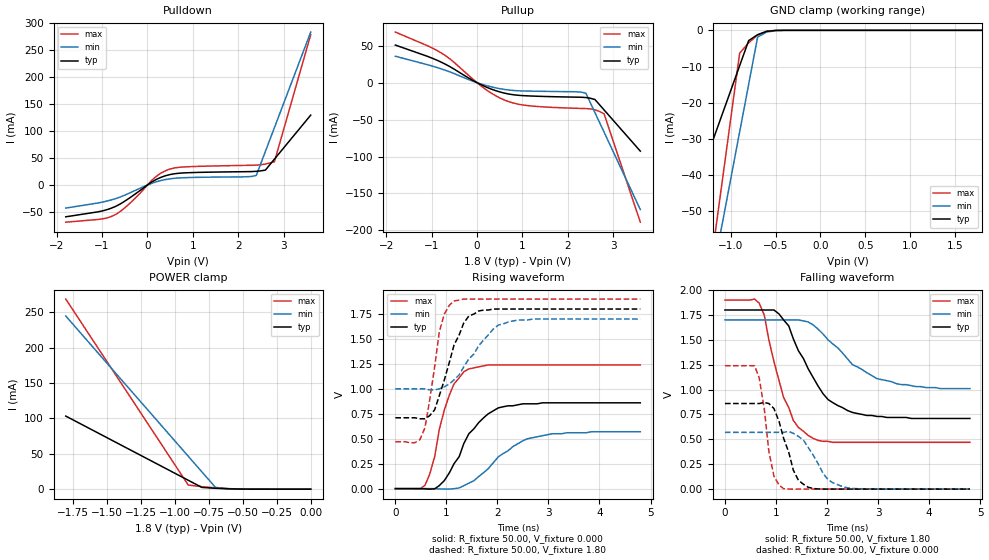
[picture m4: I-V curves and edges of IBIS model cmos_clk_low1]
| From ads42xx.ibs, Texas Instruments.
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|   Model cmos_clk_low1
[Model]   cmos_clk_low1
Model_type   3-state
Polarity   Non-Inverting
Vmeas = 1.0000V
Enable   Active-High
C_comp   5.00pF   2.00pF   8.00pF
[Temperature Range]   25.00   0.12k   -40.00
[Voltage Range]   1.80V   1.70V   1.90V
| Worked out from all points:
|   slope of the pulldown table from 0 to 0.27 V, typ, clamps not added: 20.6 ohm
|   slope of the pullup table from 0 to 0.27 V, typ, clamps not added: 35.4 ohm
|   GND clamp passes 1 mA (typ) near -0.68 V on its own axis
|   POWER clamp passes 1 mA (typ) near -0.67 V on its own axis
|   rising waveform, R_fixture 50.00, V_fixture 0.000: 20-80 % time 614ps typ, 803ps min, 373ps max; typ from 0 V to 0.86 V
|   rising waveform, R_fixture 50.00, V_fixture 1.80: 20-80 % time 423ps typ, 603ps min, 256ps max; typ from 0.71 V to 1.8 V
|   falling waveform, R_fixture 50.00, V_fixture 1.80: 20-80 % time 683ps typ, 937ps min, 475ps max; typ from 1.8 V to 0.71 V
|   falling waveform, R_fixture 50.00, V_fixture 0.000: 20-80 % time 304ps typ, 407ps min, 202ps max; typ from 0.86 V to 0 V
[Pulldown]
| voltage   I(typ)   I(min)   I(max)
-1.8V     -58.78mA   -42.68mA   -68.73mA
-1V       -48.05mA   -31.73mA   -62.68mA
-700mV    -39.48mA   -25.15mA   -54.48mA
-300mV    -18.48mA   -11.25mA   -26.98mA
200mV     10.49mA    6.06mA     16.29mA
500mV     19.33mA    11.46mA    29.59mA
900mV     22.7mA     13.73mA    33.77mA
2.2V      24.65mA    15.28mA    36.32mA
2.4V      25.28mA    17.69mA    36.7mA
2.6V      27.5mA     61.83mA    38.72mA
2.8V      47.82mA    106mA      43mA
3.6V      129.1mA    282.5mA    277.8mA
[Pullup]
| voltage   I(typ)   I(min)   I(max)
-1.8V     50.96mA    35.82mA    68.54mA
-800mV    28.12mA    18.93mA    40.73mA
-600mV    21.83mA    14.64mA    32.36mA
100mV     -3.09mA    -2.01mA    -4.98mA
400mV     -10.58mA   -6.86mA    -17.33mA
600mV     -14.08mA   -9.1mA     -23.36mA
1.1V      -17.8mA    -11.34mA   -30.94mA
2.2V      -19.61mA   -12.37mA   -34.71mA
2.4V      -20.1mA    -14.27mA   -35.09mA
2.6V      -22.83mA   -40.55mA   -36.71mA
2.8V      -36.81mA   -66.83mA   -42.02mA
3.6V      -92.73mA   -171.9mA   -189mA
[GND_clamp]
| voltage   I(typ)   I(min)   I(max)
-1.8V     -72.05mA   -145.9mA   -170.5mA
-1.6V     -58.21mA   -119.7mA   -134mA
-1.5V     -51.29mA   -106.6mA   -115.8mA
-1.2V     -30.53mA   -67.33mA   -61.04mA
-1.1V     -23.61mA   -54.24mA   -42.8mA
-1V       -16.69mA   -41.15mA   -24.56mA
-900mV    -9.77mA    -28.06mA   -6.32mA
-800mV    -2.85mA    -14.97mA   -3.46mA
-700mV    -1.2mA     -1.88mA    -1.32mA
-600mV    -300uA     -470uA     -220uA
-400mV    -2.19uA    -13.33uA   -400nA
1.8V      30.61pA    20.27nA    23.42pA
[POWER_clamp]
| voltage   I(typ)   I(min)   I(max)
-1.8V     103.3mA    244.7mA    268.7mA
-900mV    12.58mA    46.54mA    5.82mA
-800mV    2.5mA      24.52mA    3.54mA
-700mV    1.23mA     2.5mA      1.83mA
-500mV    85.21uA    200uA      92.55uA
0V        30.61pA    840pA      26.65pA
[Ramp]
| variable   typ   min   max
dV/dt_r   0.52/0.58n   0.34/0.80n   0.74/0.39n
dV/dt_f   0.65/0.70n   0.42/0.94n   0.86/0.47n
R_load = 50.00
[Rising Waveform]
R_fixture = 50.00
V_fixture = 0.000
V_fixture_min = 0.000
V_fixture_max = 0.000
| time   V(typ)   V(min)   V(max)
0s        440pV      26.42nV    250pV
580ps     -2.53mV    530uV      33.44mV
770ps     -2.3mV     -810uV     320mV
860ps     30.03mV    -3.05mV    590mV
1.06ns    160mV      -4.45mV    940mV
1.15ns    250mV      -660uV     1.05V
1.44ns    550mV      54.89mV    1.2V
2.02ns    810mV      320mV      1.24V
2.59ns    850mV      500mV      1.24V
4.8ns     860mV      570mV      1.24V
[Rising Waveform]
R_fixture = 50.00
V_fixture = 1.80
V_fixture_min = 1.70
V_fixture_max = 1.90
| time   V(typ)   V(min)   V(max)
0s        710mV      1V         470mV
380ps     710mV      1V         460mV
580ps     700mV      1V         610mV
770ps     790mV      990mV      1.22V
860ps     930mV      1V         1.57V
960ps     1.09V      1.02V      1.75V
1.15ns    1.44V      1.09V      1.88V
1.44ns    1.73V      1.3V       1.9V
2.02ns    1.8V       1.64V      1.9V
4.8ns     1.8V       1.7V       1.9V
[Falling Waveform]
R_fixture = 50.00
V_fixture = 1.80
V_fixture_min = 1.70
V_fixture_max = 1.90
| time   V(typ)   V(min)   V(max)
0s        1.8V       1.7V       1.9V
670ps     1.8V       1.7V       1.87V
770ps     1.8V       1.7V       1.75V
960ps     1.8V       1.7V       1.28V
1.15ns    1.7V       1.7V       920mV
1.34ns    1.51V      1.7V       690mV
1.73ns    1.12V      1.65V      510mV
2.11ns    870mV      1.46V      470mV
2.98ns    730mV      1.11V      470mV
4.8ns     710mV      1.01V      470mV
[Falling Waveform]
R_fixture = 50.00
V_fixture = 0.000
V_fixture_min = 0.000
V_fixture_max = 0.000
| time   V(typ)   V(min)   V(max)
0s        860mV      570mV      1.24V
580ps     860mV      570mV      1.24V
670ps     860mV      570mV      1.12V
960ps     810mV      570mV      130mV
1.15ns    510mV      570mV      3.87mV
1.34ns    190mV      560mV      -920uV
1.63ns    18.51mV    420mV      -3.19uV
2.02ns    140uV      94.59mV    840nV
2.3ns     150uV      25.49mV    -320nV
4.8ns     18.84nV    11.1uV     210pV
